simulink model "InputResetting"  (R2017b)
settings: Solver=ode15s  StartTime=0.0  StopTime=25000  MaxStep=0.1  RelTol=1e-5
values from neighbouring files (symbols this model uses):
  d = Tin_c(i)    [ActiveConstraints.m]    (also in Main.m = 293.15)
  Kc_c = 0    [ActiveConstraints.m]    (also in Main.m = -0.055)
  Kc_h_IR = 0.1    [Main.m]
  N = 10    [ActiveConstraints.m]    (also in Main.m; SRC_ODE.m = p(8))
  p = [rho_c; rho_h; Tin_h; U; A; cp_c; cp_h;N;F_c_max;F_h_max]    [ActiveConstraints.m]    (also in Main.m)
  tauI_c = 1    [ActiveConstraints.m]    (also in Main.m = 74)
  tauI_h_IR = 77    [Main.m]
  ThSP = x0(end)    [ActiveConstraints.m]    (also in Main.m)
  x0 = [Tc0; Th0]    [ActiveConstraints.m]    (also in Main.m; col_obj.m = 0.5*ones(1,82)'; Simulate1Col.m = x; Simulate1Col_OL.m = x)
  z_c = F_c/F_c_max    (= 1)    [ActiveConstraints.m]    (also in Main.m = 0.5; SRC_ODE.m = u(1))
  z_h = F_h./F_h_max    [ActiveConstraints.m]    (also in Main.m = 1; SRC_ODE.m = u(2))
undefined symbols (not defined in the file or in its folder): SRC_ODE
libraries: simulink x2

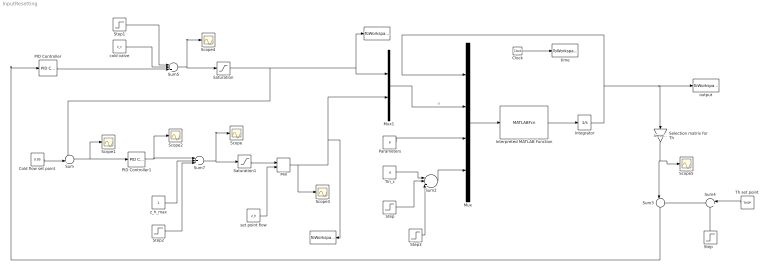
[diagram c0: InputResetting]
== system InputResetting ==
  " " : ToWorkspace  VariableName=u1  SampleTime=-1
  "  " : ToWorkspace  VariableName=u2  SampleTime=-1
  Clock : Clock
  Cold flow set point : Constant  Value=0.95
  Integrator : Integrator  InitialCondition=x0'
  Interpreted MATLAB Function : MATLABFcn  MATLABFcn=SRC_ODE(u(1:20),u(21:22),u(23:32),u(33))  OutputDimensions=20  Output1D=off
  Min : MinMax  Inputs=2
  Mux : Mux
  Mux1 : Mux  Inputs=2
  PID Controller : simulink/Continuous/PID Controller  Controller=PI  TimeDomain=Continuous-time  SampleTime=-1  IntegratorMethod=Forward Euler  FilterMethod=Forward Euler  Form=Parallel  UseFilter=on  ControllerParametersSource=internal  P=Kc_c  I=Kc_c/tauI_c  D=0  N=100  InitialConditionSource=internal  InitialConditionForIntegrator=0  InitialConditionForFilter=0  ExternalReset=none  IgnoreLimit=on  ZeroCross=off  LimitOutput=off  UpperSaturationLimit=1  LowerSaturationLimit=0  LinearizeAsGain=on  AntiWindupMode=back-calculation  Kb=1  TrackingMode=off  Kt=1  PParamMin=[]  PParamMax=[]  IParamMin=[]  IParamMax=[]  DParamMin=[]  DParamMax=[]  NParamMin=[]  NParamMax=[]  KbParamMin=[]  KbParamMax=[]  KtParamMin=[]  KtParamMax=[]  POutMin=[]  POutMax=[]  IOutMin=[]  IOutMax=[]  DOutMin=[]  DOutMax=[]  NOutMin=[]  NOutMax=[]  KbOutMin=[]  KbOutMax=[]  KtOutMin=[]  KtOutMax=[]  IntegratorOutMin=[]  IntegratorOutMax=[]  FilterOutMin=[]  FilterOutMax=[]  SumOutMin=[]  SumOutMax=[]  SumI1OutMin=[]  SumI1OutMax=[]  SumI2OutMin=[]  SumI2OutMax=[]  SumI3OutMin=[]  SumI3OutMax=[]  SumDOutMin=[]  SumDOutMax=[]  SaturationOutMin=[]  SaturationOutMax=[]  IntegratorContinuousStateAttributes=''  IntegratorStateMustResolveToSignalObject=off  IntegratorRTWStateStorageClass=Auto  FilterContinuousStateAttributes=''  FilterStateMustResolveToSignalObject=off  FilterRTWStateStorageClass=Auto  DifferentiatorICPrevScaledInput=0  DifferentiatorOutMin=[]  DifferentiatorOutMax=[]  InitialConditionSetting=State (most efficient)  FilterDiffOutCoefMin=[]  FilterDiffOutCoefMax=[]  SumDenOutMin=[]  SumDenOutMax=[]  SumNumOutMin=[]  SumNumOutMax=[]  ReciprocalOutMin=[]  ReciprocalOutMax=[]  DivideOutMin=[]  DivideOutMax=[]  TunerSelectOption=Transfer Function Based (PID Tuner App)
  PID Controller1 : simulink/Continuous/PID Controller  Controller=PI  TimeDomain=Continuous-time  SampleTime=-1  IntegratorMethod=Forward Euler  FilterMethod=Forward Euler  Form=Parallel  UseFilter=on  ControllerParametersSource=internal  P=Kc_h_IR  I=Kc_h_IR/tauI_h_IR  D=0  N=100  InitialConditionSource=internal  InitialConditionForIntegrator=0  InitialConditionForFilter=0  ExternalReset=none  LimitOutput=on  UpperSaturationLimit=0  LowerSaturationLimit=-1  LinearizeAsGain=on  AntiWindupMode=back-calculation  Kb=100  TrackingMode=off  Kt=1  PParamMin=[]  PParamMax=[]  IParamMin=[]  IParamMax=[]  DParamMin=[]  DParamMax=[]  NParamMin=[]  NParamMax=[]  KbParamMin=[]  KbParamMax=[]  KtParamMin=[]  KtParamMax=[]  POutMin=[]  POutMax=[]  IOutMin=[]  IOutMax=[]  DOutMin=[]  DOutMax=[]  NOutMin=[]  NOutMax=[]  KbOutMin=[]  KbOutMax=[]  KtOutMin=[]  KtOutMax=[]  IntegratorOutMin=[]  IntegratorOutMax=[]  FilterOutMin=[]  FilterOutMax=[]  SumOutMin=[]  SumOutMax=[]  SumI1OutMin=[]  SumI1OutMax=[]  SumI2OutMin=[]  SumI2OutMax=[]  SumI3OutMin=[]  SumI3OutMax=[]  SumDOutMin=[]  SumDOutMax=[]  SaturationOutMin=[]  SaturationOutMax=[]  IntegratorContinuousStateAttributes=''  IntegratorStateMustResolveToSignalObject=off  IntegratorRTWStateStorageClass=Auto  FilterContinuousStateAttributes=''  FilterStateMustResolveToSignalObject=off  FilterRTWStateStorageClass=Auto  DifferentiatorICPrevScaledInput=0  DifferentiatorOutMin=[]  DifferentiatorOutMax=[]  InitialConditionSetting=State (most efficient)  FilterDiffOutCoefMin=[]  FilterDiffOutCoefMax=[]  SumDenOutMin=[]  SumDenOutMax=[]  SumNumOutMin=[]  SumNumOutMax=[]  ReciprocalOutMin=[]  ReciprocalOutMax=[]  DivideOutMin=[]  DivideOutMax=[]  TunerSelectOption=Transfer Function Based (PID Tuner App)
  Parameters : Constant  Value=p
  Saturation : Saturate  UpperLimit=1  LowerLimit=0
  Saturation1 : Saturate  UpperLimit=1  LowerLimit=0
  Scope{,1..5} (6 alike) : Scope
  Selection matrix for Th : Gain  Gain=[zeros(1,2*N-1),1]  Multiplication=Matrix(K*u)
  Step : Step  Time=200  After=2  SampleTime=0
  "Step   " : Step  Time=50  After=0  SampleTime=0
  Step1 : Step  Time=0  After=0  SampleTime=0
  Step2 : Step  Time=100  After=0  SampleTime=0
  Step3 : Step  Time=2000  After=4  SampleTime=0
  Sum : Sum  Inputs=-+|
  Sum2 : Sum  Inputs=|+++
  Sum3 : Sum  Inputs=|-+
  Sum4 : Sum  Inputs=|++
  Sum5 : Sum  Inputs=+++|
  Sum7 : Sum  Inputs=|+++
  Th set point : Constant  Value=ThSP
  Tin_c : Constant  Value=d
  cold valve : Constant  Value=z_c
  output : ToWorkspace  VariableName=y  SampleTime=-1
  set point flow : Constant  Value=z_h
  time : ToWorkspace  VariableName=t  SampleTime=-1
  z_h_max : Constant
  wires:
  Interpreted MATLAB Function/1 -> Integrator/1
  Mux/1 -> Interpreted MATLAB Function/1
  Clock/1 -> time/1
  Mux1/1 -> Mux/2  "u"
  Parameters/1 -> Mux/3
  Tin_c/1 -> Sum2/1
  Step/1 -> Sum2/2
  Sum2/1 -> Mux/4
  Sum4/1 -> Sum3/2
  "Step   "/1 -> Sum4/2
  Th set point/1 -> Sum4/1
  Sum3/1 -> PID Controller/1
  z_h_max/1 -> Sum7/2
  Saturation/1 -> Sum/1, Mux1/1, " "/1
  Sum5/1 -> Scope4/1, Saturation/1
  Saturation1/1 -> Min/1
  Sum7/1 -> Scope/1, Saturation1/1
  set point flow/1 -> Min/2
  Min/1 -> Scope3/1, "  "/1, Mux1/2
  PID Controller/1 -> Sum5/3
  cold valve/1 -> Sum5/2
  Step1/1 -> Sum5/1
  Sum/1 -> Scope1/1, PID Controller1/1
  PID Controller1/1 -> Scope2/1, Sum7/1
  Cold flow set point/1 -> Sum/2
  Step2/1 -> Sum7/3
  Step3/1 -> Sum2/3
  Selection matrix for Th/1 -> Sum3/1, Scope5/1
  Integrator/1 -> Selection matrix for Th/1, output/1, Mux/1
